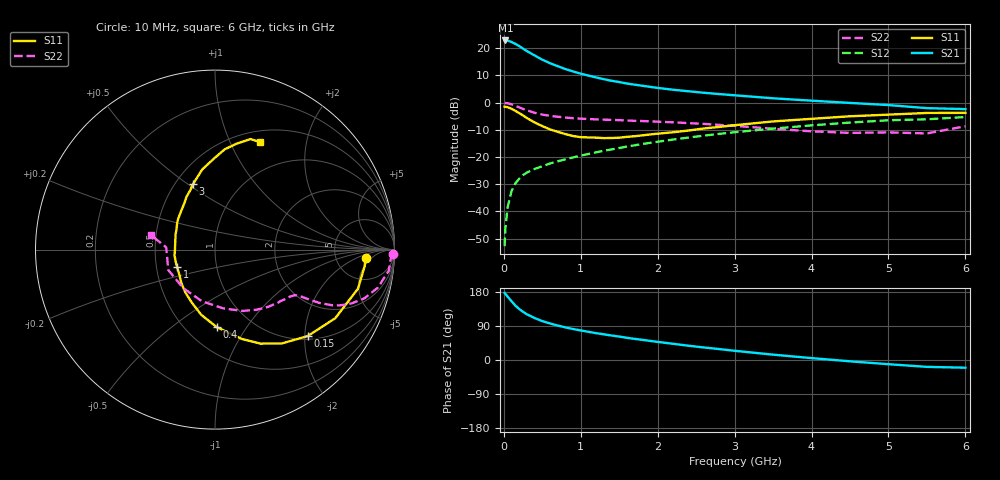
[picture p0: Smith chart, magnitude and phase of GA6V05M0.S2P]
! Infineon Technologies  Discrete & RF Semiconductors
! BF775
! Si NPN RF Bipolar Junction Transistor in SOT23
! VCE = 6 V  IC = 5 mA
! Common Emitter S-Parameters:  May  1996
# GHz  S  MA  R  50
!  f  S11  S21  S12  S22
! GHz  MAG  ANG  MAG  ANG  MAG  ANG  MAG  ANG
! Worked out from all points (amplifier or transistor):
!   36 points, 10 MHz to 6 GHz, reference 50 ohm
!   highest |S21| = 22.9 dB at 20 MHz (marker M1)
!   |S21| within 3 dB of that: start of sweep to 248.5 MHz
!   unconditionally stable (mu >= 1): 834.6 MHz to 3.085 GHz
!   at 250 MHz: K = 0.48, MSG = 23.2 dB, |S12| = -26.6 dB
!   at 1.4 GHz: K = 1.11, MAG = 10.6 dB, |S12| = -17.2 dB
!   at 6 GHz: K = 0.92, MSG = 1.5 dB, |S12| = -5.3 dB
!   lowest NFmin = 1.50 dB at 450 MHz
!   S11 on the Smith chart (normalised r, x): 10 MHz: 11, -3; 150 MHz: 1.08, -2.07; 400 MHz: 0.70, -0.74; 1 GHz: 0.64, -0.13; 3 GHz: 0.61, +0.52; 6 GHz: 0.63, +1.30
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0.01  0.8416 -3.1  13.88 177.3  0.0023 90.9  0.9934 -1.3
0.02  0.839 -6.3  13.92 174.4  0.0049 88.7  0.9814 -2.7
0.05  0.8259 -15.3  13.84 167.0  0.0121 82.0  0.9752 -6.9
0.1  0.7714 -29.7  13.01 155.1  0.0237 74.8  0.9323 -13.1
0.15  0.7063 -43.0  12.04 143.5  0.0328 68.8  0.8763 -18.0
0.2  0.6417 -54.6  10.98 134.6  0.04 65.0  0.8179 -21.5
0.25  0.5819 -64.2  9.821 127.0  0.0467 61.2  0.766 -23.9
0.3  0.5204 -73.2  8.881 120.6  0.052 59.8  0.7235 -25.4
0.4  0.4326 -88.6  7.376 110.8  0.0604 57.8  0.6513 -27.1
0.5  0.3708 -102.0  6.158 102.7  0.0678 57.1  0.603 -27.8
0.6  0.3231 -113.4  5.322 96.4  0.0761 57.3  0.5733 -28.2
0.8  0.2645 -135.1  4.152 86.1  0.0909 57.7  0.5332 -28.9
1  0.2325 -155.3  3.409 78.0  0.1061 58.9  0.5083 -30.1
1.1  0.2293 -163.1  3.143 74.4  0.114 59.0  0.5002 -31.2
1.3  0.2232 -179.8  2.699 67.8  0.1307 58.9  0.487 -33.2
1.6  0.2352 159.1  2.25 58.5  0.1557 58.4  0.4697 -37.0
2.2  0.2857 131.4  1.729 42.8  0.2098 55.5  0.4353 -47.0
3  0.3851 108.5  1.366 24.3  0.2861 48.6  0.3749 -65.7
3.5  0.4519 99.1  1.203 14.1  0.3336 43.2  0.3307 -82.0
4.5  0.562 84.4  0.989 -3.5  0.4309 30.9  0.2781 -129.8
5.5  0.647 72.2  0.793 -18.1  0.4945 15.6  0.272 177.4
6  0.6491 67.2  0.761 -20.3  0.5444 11.4  0.3679 167.0
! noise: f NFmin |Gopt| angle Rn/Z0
0.45  1.5  0.28  29  0.34
0.9  1.8  0.25  59  0.34
